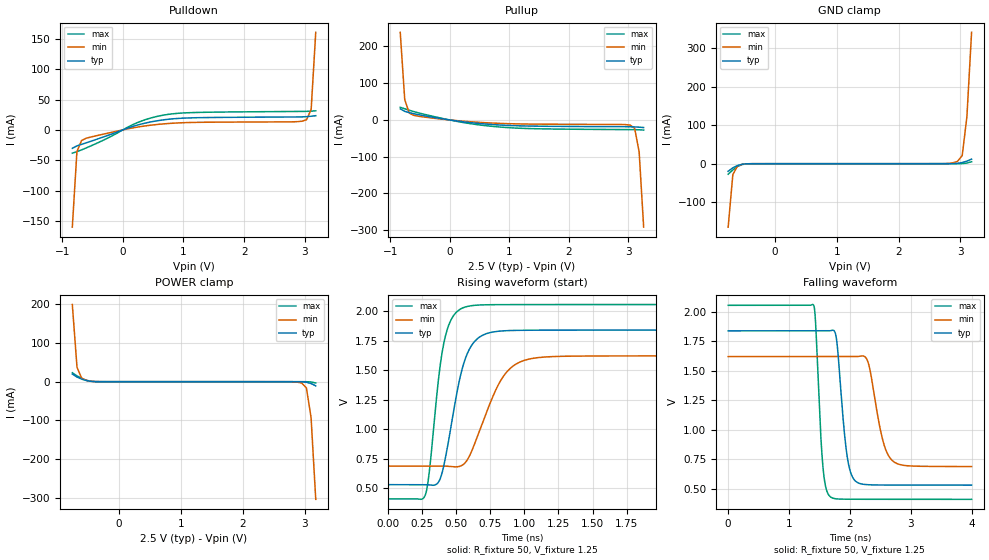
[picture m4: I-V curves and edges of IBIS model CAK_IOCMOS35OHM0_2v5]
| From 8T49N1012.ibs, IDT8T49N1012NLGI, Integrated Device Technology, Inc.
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| 3.25758e+00   -1.33581e-02   -4.69445e-01   -6.92786e-03
| 3.33333e+00   -3.05431e-02   -6.81022e-01   -1.35814e-02
| 3.40909e+00   -1.97473e-01   -8.92821e-01   -2.11713e-02
| 3.48485e+00   -4.80532e-01   -1.10478e+00   -2.82326e-02
| 3.56061e+00   -7.63803e-01   -1.31687e+00   -5.48408e-02
| 3.63636e+00   -1.04727e+00   -1.52909e+00   -3.40378e-01
| 3.71212e+00   -1.33091e+00   -1.74141e+00   -7.03030e-01
| 3.78788e+00   -1.61471e+00   -1.95383e+00   -1.06588e+00
| 3.86364e+00   -1.89867e+00   -2.16636e+00   -1.42892e+00
| 3.93939e+00   -2.18277e+00   -2.37898e+00   -1.79210e+00
| 4.01515e+00   -2.46699e+00   -2.59169e+00   -2.15542e+00
| 4.09091e+00   -2.75133e+00   -2.80449e+00   -2.51885e+00
| 4.16667e+00   -3.03577e+00   -3.01738e+00   -2.88238e+00
| 4.24242e+00   -3.32030e+00   -3.23034e+00   -3.24599e+00
| 4.31818e+00   -3.60492e+00   -3.44338e+00   -3.60966e+00
| 4.39394e+00   -3.88961e+00   -3.65649e+00   -3.97340e+00
| 4.46970e+00   -4.17436e+00   -3.86967e+00   -4.33720e+00
| 4.54545e+00   -4.45918e+00   -4.08291e+00   -4.70105e+00
| 4.62121e+00   -4.74404e+00   -4.29621e+00   -5.06495e+00
| 4.69697e+00   -5.02895e+00   -4.50957e+00   -5.42889e+00
| 4.77273e+00   -5.31390e+00   -4.72298e+00   -5.79286e+00
| 4.84848e+00   -5.59889e+00   -4.93644e+00   -6.15686e+00
| 4.92424e+00   -5.88390e+00   -5.14994e+00   -6.52088e+00
| 5.00000e+00   -6.16895e+00   -5.36349e+00   -6.88491e+00
[Model] CAK_IOCMOS35OHM0_2v5
Model_type   I/O
Polarity   Non-Inverting
|   typ   min   max
C_comp   2pF   1.5pF   2.5pF
|Input
Vinl = 0.7V
Vinh = 1.7V
|Output
Vmeas = 1.25V
Rref = 50
Cref = 0
Vref = 1.25V
|   typ   min   max
[Voltage range]   2.5V   2.375V   2.625V
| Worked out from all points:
|   slope of the pulldown table from 0 to 0.375 V, typ, clamps not added: 33.2 ohm
|   slope of the pullup table from 0 to 0.375 V, typ, clamps not added: 48.8 ohm
|   GND clamp passes 1 mA (typ) near -0.50 V on its own axis
|   POWER clamp passes 1 mA (typ) near -0.46 V on its own axis
|   rising waveform, R_fixture 50, V_fixture 1.25: 20-80 % time 134ps typ, 204ps min, 96.8ps max; typ from 0.531 V to 1.84 V
|   falling waveform, R_fixture 50, V_fixture 1.25: 20-80 % time 134ps typ, 204ps min, 95ps max; typ from 1.84 V to 0.531 V
[GND_clamp]
|Voltage   I (typ)   I (min)   I (max)
|Note, modeling breaks down at 250mA and above.  This is well beyond the functional   |
|operating range of the device.  Should this scenario occur, catastrophic failure and   |
|possible damage to the device and/or board is of higher concern than the I-V curve   |
|behavior.  The IBIS checker will flag currents in excess of 10A with warnings.  Lines   |
|with currents in excess of 0.35 A have been commented out.  The points still remain|
|available to the user if the user desires to use them.   |
|-2.42424e+00   -5.99088e+00   -4.88415e+00   -7.24880e+00
|-2.34848e+00   -5.70272e+00   -4.66840e+00   -6.88094e+00
|-2.27273e+00   -5.41462e+00   -4.45272e+00   -6.51310e+00
|-2.19697e+00   -5.12656e+00   -4.23712e+00   -6.14529e+00
|-2.12121e+00   -4.83856e+00   -4.02161e+00   -5.77750e+00
|-2.04545e+00   -4.55064e+00   -3.80620e+00   -5.40975e+00
|-1.96970e+00   -4.26278e+00   -3.59088e+00   -5.04205e+00
|-1.89394e+00   -3.97502e+00   -3.37567e+00   -4.67441e+00
|-1.81818e+00   -3.68735e+00   -3.16057e+00   -4.30683e+00
|-1.74242e+00   -3.39979e+00   -2.94558e+00   -3.93934e+00
|-1.66667e+00   -3.11235e+00   -2.73072e+00   -3.57193e+00
|-1.59091e+00   -2.82505e+00   -2.51599e+00   -3.20462e+00
|-1.51515e+00   -2.53790e+00   -2.30139e+00   -2.83743e+00
|-1.43939e+00   -2.25092e+00   -2.08694e+00   -2.47036e+00
|-1.36364e+00   -1.96413e+00   -1.87263e+00   -2.10344e+00
|-1.28788e+00   -1.67754e+00   -1.65847e+00   -1.73670e+00
|-1.21212e+00   -1.39118e+00   -1.44447e+00   -1.37017e+00
|-1.13636e+00   -1.10506e+00   -1.23064e+00   -1.00389e+00
|-1.06061e+00   -8.19198e-01   -1.01701e+00   -6.37879e-01
|-9.84848e-01   -5.33627e-01   -8.03591e-01   -2.72184e-01
|-9.09091e-01   -2.48371e-01   -5.90465e-01   -5.58283e-02
|-8.33333e-01   -4.53732e-02   -3.77762e-01   -3.79192e-02
-757.6mV  -19.7mA    -165.1mA   -27.4mA
-681.8mV  -10.83mA   -28.37mA   -16.29mA
-606.1mV  -4.786mA   -6.047mA   -7.399mA
-530.3mV  -1.407mA   -1.506mA   -2.105mA
-378.8mV  -80.75uA   -97.08uA   -91.06uA
2.727V    4.903uA    107uA      2.354uA
2.879V    114.3uA    2.196mA    6.393uA
2.955V    801.8uA    6.121mA    22.36uA
3.03V     2.877mA    21.15mA    238.2uA
3.106V    6.558mA    121.9mA    1.646mA
3.182V    11.89mA    341.6mA    5.038mA
| 3.25758e+00   1.96472e-02   5.60110e-01   1.04123e-02
| 3.33333e+00   4.87507e-02   7.78570e-01   1.76749e-02
| 3.40909e+00   2.77107e-01   9.97201e-01   2.56783e-02
| 3.48485e+00   5.68788e-01   1.21604e+00   3.28468e-02
| 3.56061e+00   8.60732e-01   1.43508e+00   7.83400e-02
| 3.63636e+00   1.15296e+00   1.65434e+00   4.20975e-01
| 3.71212e+00   1.44548e+00   1.87382e+00   7.94432e-01
| 3.78788e+00   1.73828e+00   2.09351e+00   1.16825e+00
| 3.86364e+00   2.03137e+00   2.31341e+00   1.54243e+00
| 3.93939e+00   2.32473e+00   2.53352e+00   1.91695e+00
| 4.01515e+00   2.61836e+00   2.75385e+00   2.29181e+00
| 4.09091e+00   2.91225e+00   2.97438e+00   2.66701e+00
| 4.16667e+00   3.20641e+00   3.19513e+00   3.04252e+00
| 4.24242e+00   3.50082e+00   3.41608e+00   3.41834e+00
| 4.31818e+00   3.79548e+00   3.63725e+00   3.79446e+00
| 4.39394e+00   4.09039e+00   3.85863e+00   4.17087e+00
| 4.46970e+00   4.38554e+00   4.08023e+00   4.54756e+00
| 4.54545e+00   4.68094e+00   4.30204e+00   4.92452e+00
| 4.62121e+00   4.97658e+00   4.52407e+00   5.30175e+00
| 4.69697e+00   5.27245e+00   4.74633e+00   5.67924e+00
| 4.77273e+00   5.56857e+00   4.96881e+00   6.05699e+00
| 4.84848e+00   5.86492e+00   5.19152e+00   6.43499e+00
| 4.92424e+00   6.16151e+00   5.41446e+00   6.81323e+00
| 5.00000e+00   6.45834e+00   5.63765e+00   7.19172e+00
[Power_clamp]
|Voltage   I (typ)   I (min)   I (max)
|Note, modeling breaks down at 250mA and above.  This is well beyond the functional   |
|operating range of the device.  Should this scenario occur, catastrophic failure and   |
|possible damage to the device and/or board is of higher concern than the I-V curve   |
|behavior.  The IBIS checker will flag currents in excess of 10A with warnings.  Lines   |
|with currents in excess of 0.35 A have been commented out.  The points still remain|
|available to the user if the user desires to use them.   |
|-2.42424e+00   6.16151e+00   5.04673e+00   7.43787e+00
|-2.34848e+00   5.86492e+00   4.82417e+00   7.05922e+00
|-2.27273e+00   5.56857e+00   4.60184e+00   6.68082e+00
|-2.19697e+00   5.27245e+00   4.37973e+00   6.30266e+00
|-2.12121e+00   4.97658e+00   4.15784e+00   5.92475e+00
|-2.04545e+00   4.68094e+00   3.93617e+00   5.54709e+00
|-1.96970e+00   4.38554e+00   3.71471e+00   5.16969e+00
|-1.89394e+00   4.09039e+00   3.49347e+00   4.79255e+00
|-1.81818e+00   3.79548e+00   3.27244e+00   4.41568e+00
|-1.74242e+00   3.50082e+00   3.05162e+00   4.03909e+00
|-1.66667e+00   3.20641e+00   2.83101e+00   3.66278e+00
|-1.59091e+00   2.91225e+00   2.61061e+00   3.28677e+00
|-1.51515e+00   2.61836e+00   2.39042e+00   2.91105e+00
|-1.43939e+00   2.32473e+00   2.17045e+00   2.53565e+00
|-1.36364e+00   2.03137e+00   1.95069e+00   2.16057e+00
|-1.28788e+00   1.73828e+00   1.73114e+00   1.78583e+00
|-1.21212e+00   1.44548e+00   1.51180e+00   1.41142e+00
|-1.13636e+00   1.15296e+00   1.29268e+00   1.03737e+00
|-1.06061e+00   8.60732e-01   1.07377e+00   6.63681e-01
|-9.84848e-01   5.68788e-01   8.55069e-01   2.90350e-01
|-9.09091e-01   2.77107e-01   6.36557e-01   4.68087e-02
|-8.33333e-01   4.87507e-02   4.18123e-01   3.00765e-02
-757.6mV  19.65mA    199mA      23mA
-681.8mV  11.89mA    37.01mA    14.94mA
-606.1mV  6.558mA    8.981mA    8.308mA
-530.3mV  2.877mA    3.169mA    3.622mA
-303mV    14.46uA    30.61uA    12.18uA
2.727V    -54.42uA   -72.56uA   -62.76uA
2.879V    -80.75uA   -908.8uA   -66.34uA
2.955V    -281.2uA   -3.717mA   -70.88uA
3.03V     -1.407mA   -15.93mA   -127.8uA
3.106V    -4.786mA   -92.25mA   -684.1uA
3.182V    -10.83mA   -303.4mA   -3.499mA
| 3.25758e+00   -1.96989e-02   -5.15962e-01   -1.01554e-02
| 3.33333e+00   -4.53732e-02   -7.28958e-01   -2.00234e-02
| 3.40909e+00   -2.48371e-01   -9.42283e-01   -3.12866e-02
| 3.48485e+00   -5.33627e-01   -1.15585e+00   -4.17513e-02
| 3.56061e+00   -8.19198e-01   -1.36961e+00   -8.15325e-02
| 3.63636e+00   -1.10506e+00   -1.58355e+00   -4.00139e-01
| 3.71212e+00   -1.39118e+00   -1.79765e+00   -7.65947e-01
| 3.78788e+00   -1.67754e+00   -2.01191e+00   -1.13206e+00
| 3.86364e+00   -1.96413e+00   -2.22632e+00   -1.49843e+00
| 3.93939e+00   -2.25092e+00   -2.44086e+00   -1.86504e+00
| 4.01515e+00   -2.53790e+00   -2.65555e+00   -2.23184e+00
| 4.09091e+00   -2.82505e+00   -2.87037e+00   -2.59881e+00
| 4.16667e+00   -3.11235e+00   -3.08531e+00   -2.96593e+00
| 4.24242e+00   -3.39979e+00   -3.30037e+00   -3.33317e+00
| 4.31818e+00   -3.68735e+00   -3.51555e+00   -3.70052e+00
| 4.39394e+00   -3.97502e+00   -3.73083e+00   -4.06795e+00
| 4.46970e+00   -4.26278e+00   -3.94621e+00   -4.43548e+00
| 4.54545e+00   -4.55064e+00   -4.16168e+00   -4.80307e+00
| 4.62121e+00   -4.83856e+00   -4.37725e+00   -5.17074e+00
| 4.69697e+00   -5.12656e+00   -4.59290e+00   -5.53846e+00
| 4.77273e+00   -5.41462e+00   -4.80863e+00   -5.90622e+00
| 4.84848e+00   -5.70272e+00   -5.02443e+00   -6.27402e+00
| 4.92424e+00   -5.99088e+00   -5.24031e+00   -6.64184e+00
| 5.00000e+00   -6.27908e+00   -5.45625e+00   -7.00969e+00
[Pulldown]
|Voltage   I (typ)   I (min)   I (max)
|Note, modeling breaks down at 250mA and above.  This is well beyond the functional   |
|operating range of the device.  Should this scenario occur, catastrophic failure and   |
|possible damage to the device and/or board is of higher concern than the I-V curve   |
|behavior.  The IBIS checker will flag currents in excess of 10A with warnings.  Lines   |
|with currents in excess of 0.35 A have been commented out.  The points still remain|
|available to the user if the user desires to use them.   |
|-2.424240e+00   -5.620920e+00   -4.561270e+00   -6.831600e+00
|-2.348480e+00   -5.341380e+00   -4.351820e+00   -6.474360e+00
|-2.272730e+00   -5.061780e+00   -4.142370e+00   -6.117000e+00
|-2.196970e+00   -4.782250e+00   -3.932930e+00   -5.759610e+00
|-2.121210e+00   -4.502700e+00   -3.723470e+00   -5.402300e+00
|-2.045450e+00   -4.223130e+00   -3.514010e+00   -5.044950e+00
|-1.969700e+00   -3.943570e+00   -3.304540e+00   -4.687600e+00
|-1.893940e+00   -3.663980e+00   -3.095070e+00   -4.330220e+00
|-1.818180e+00   -3.384390e+00   -2.885580e+00   -3.972840e+00
|-1.742420e+00   -3.104780e+00   -2.676080e+00   -3.615430e+00
|-1.666670e+00   -2.825150e+00   -2.466570e+00   -3.258010e+00
|-1.590910e+00   -2.545490e+00   -2.257030e+00   -2.900560e+00
|-1.515150e+00   -2.265810e+00   -2.047480e+00   -2.543070e+00
|-1.439390e+00   -1.986090e+00   -1.837900e+00   -2.185550e+00
|-1.363640e+00   -1.706320e+00   -1.628300e+00   -1.827980e+00
|-1.287880e+00   -1.426520e+00   -1.418670e+00   -1.470360e+00
|-1.212120e+00   -1.146650e+00   -1.209020e+00   -1.112660e+00
|-1.136360e+00   -8.667200e-01   -9.993300e-01   -7.548700e-01
|-1.060610e+00   -5.867220e-01   -7.896000e-01   -3.969910e-01
|-9.848480e-01   -3.066460e-01   -5.798390e-01   -7.806800e-02
|-9.090910e-01   -6.551900e-02   -3.700490e-01   -4.152980e-02
-833.3mV  -30.4mA    -160.2mA   -38.37mA
-757.6mV  -26.34mA   -35.84mA   -35.89mA
-681.8mV  -23.84mA   -17.61mA   -32.95mA
-606.1mV  -21.34mA   -13.8mA    -29.8mA
227.3mV   7.551mA    4.361mA    11.42mA
454.5mV   12.99mA    7.63mA     19.37mA
681.8mV   16.67mA    9.951mA    24.52mA
1.212V    20.01mA    12.36mA    28.66mA
2.803V    21.22mA    13.27mA    30.3mA
3.03V     21.8mA     16.76mA    30.5mA
3.106V    22.45mA    33.64mA    30.79mA
3.182V    23.38mA    160.7mA    31.41mA
|3.257580e+00   2.470960e-02   3.762400e-01   3.236290e-02
|3.333330e+00   2.959920e-02   5.918100e-01   3.363400e-02
|3.409090e+00   1.001510e-01   8.074090e-01   3.503170e-02
|3.484850e+00   3.838970e-01   1.023030e+00   3.629400e-02
|3.560610e+00   6.718180e-01   1.238710e+00   4.394800e-02
|3.636360e+00   9.597900e-01   1.454410e+00   2.364620e-01
|3.712120e+00   1.247810e+00   1.670150e+00   6.046980e-01
|3.787880e+00   1.535890e+00   1.885920e+00   9.730100e-01
|3.863640e+00   1.824010e+00   2.101740e+00   1.341380e+00
|3.939390e+00   2.112190e+00   2.317600e+00   1.709840e+00
|4.015150e+00   2.400420e+00   2.533480e+00   2.078370e+00
|4.090910e+00   2.688710e+00   2.749420e+00   2.446960e+00
|4.166670e+00   2.977050e+00   2.965390e+00   2.815630e+00
|4.242420e+00   3.265440e+00   3.181400e+00   3.184380e+00
|4.318180e+00   3.553900e+00   3.397450e+00   3.553210e+00
|4.393940e+00   3.842420e+00   3.613550e+00   3.922130e+00
|4.469700e+00   4.131000e+00   3.829690e+00   4.291130e+00
|4.545450e+00   4.419630e+00   4.045870e+00   4.660220e+00
|4.621210e+00   4.708340e+00   4.262110e+00   5.029450e+00
|4.696970e+00   4.997150e+00   4.478390e+00   5.398660e+00
|4.772730e+00   5.285930e+00   4.694720e+00   5.768110e+00
|4.848480e+00   5.574880e+00   4.911080e+00   6.137610e+00
|4.924240e+00   5.863890e+00   5.127540e+00   6.507170e+00
|5.000000e+00   6.153060e+00   5.344050e+00   6.876880e+00
[Pullup]
|Voltage   I (typ)   I (min)   I (max)
|Note, modeling breaks down at 250mA and above.  This is well beyond the functional   |
|operating range of the device.  Should this scenario occur, catastrophic failure and   |
|possible damage to the device and/or board is of higher concern than the I-V curve   |
|behavior.  The IBIS checker will flag currents in excess of 10A with warnings.  Lines   |
|with currents in excess of 0.35 A have been commented out.  The points still remain|
|available to the user if the user desires to use them.   |
|-2.424240e+00   5.884990e+00   4.790360e+00   7.136830e+00
|-2.348480e+00   5.595580e+00   4.573450e+00   6.766980e+00
|-2.272730e+00   5.306130e+00   4.356560e+00   6.397080e+00
|-2.196970e+00   5.016750e+00   4.139690e+00   6.027240e+00
|-2.121210e+00   4.727390e+00   3.922850e+00   5.657350e+00
|-2.045450e+00   4.438030e+00   3.706020e+00   5.287510e+00
|-1.969700e+00   4.148680e+00   3.489220e+00   4.917710e+00
|-1.893940e+00   3.859340e+00   3.272430e+00   4.547940e+00
|-1.818180e+00   3.570020e+00   3.055660e+00   4.178140e+00
|-1.742420e+00   3.280710e+00   2.838900e+00   3.808350e+00
|-1.666670e+00   2.991410e+00   2.622170e+00   3.438570e+00
|-1.590910e+00   2.702130e+00   2.405450e+00   3.068780e+00
|-1.515150e+00   2.412850e+00   2.188750e+00   2.699010e+00
|-1.439390e+00   2.123580e+00   1.972050e+00   2.329220e+00
|-1.363640e+00   1.834310e+00   1.755360e+00   1.959430e+00
|-1.287880e+00   1.545050e+00   1.538690e+00   1.589620e+00
|-1.212120e+00   1.255770e+00   1.322030e+00   1.219810e+00
|-1.136360e+00   9.665000e-01   1.105370e+00   8.499700e-01
|-1.060610e+00   6.772080e-01   8.887100e-01   4.801090e-01
|-9.848480e-01   3.878980e-01   6.720410e-01   1.143440e-01
|-9.090910e-01   1.026590e-01   4.553330e-01   3.942970e-02
-833.3mV  30.43mA    238.5mA    34.47mA
-757.6mV  23.4mA     55.15mA    30.53mA
-681.8mV  19.94mA    18.68mA    26.41mA
-606.1mV  17.11mA    12.63mA    22.8mA
151.5mV   -3.441mA   -2.312mA   -4.819mA
833.3mV   -13.62mA   -9.198mA   -19.09mA
1.439V    -16.78mA   -11.29mA   -23.78mA
2.955V    -18.33mA   -12.6mA    -26.15mA
3.03V     -18.49mA   -13.96mA   -26.22mA
3.106V    -18.9mA    -22.45mA   -26.34mA
3.182V    -19.59mA   -87.06mA   -26.7mA
3.258V    -20.6mA    -291.6mA   -27.48mA
|3.333330e+00   -2.346490e-02   -5.006320e-01   -2.861170e-02
|3.409090e+00   -5.753200e-02   -7.096670e-01   -2.989430e-02
|3.484850e+00   -2.977200e-01   -9.187300e-01   -3.108580e-02
|3.560610e+00   -5.769620e-01   -1.127830e+00   -3.553250e-02
|3.636360e+00   -8.562400e-01   -1.336930e+00   -1.541430e-01
|3.712120e+00   -1.135550e+00   -1.546060e+00   -5.113230e-01
|3.787880e+00   -1.414880e+00   -1.755200e+00   -8.685300e-01
|3.863640e+00   -1.694240e+00   -1.964350e+00   -1.225770e+00
|3.939390e+00   -1.973620e+00   -2.173530e+00   -1.583030e+00
|4.015150e+00   -2.253020e+00   -2.382720e+00   -1.940320e+00
|4.090910e+00   -2.532440e+00   -2.591920e+00   -2.297640e+00
|4.166670e+00   -2.811880e+00   -2.801140e+00   -2.654970e+00
|4.242420e+00   -3.091330e+00   -3.010380e+00   -3.012320e+00
|4.318180e+00   -3.370810e+00   -3.219620e+00   -3.369680e+00
|4.393940e+00   -3.650300e+00   -3.428890e+00   -3.727080e+00
|4.469700e+00   -3.929810e+00   -3.638170e+00   -4.084480e+00
|4.545450e+00   -4.209330e+00   -3.847470e+00   -4.441910e+00
|4.621210e+00   -4.488880e+00   -4.056780e+00   -4.799350e+00
|4.696970e+00   -4.768440e+00   -4.266100e+00   -5.156840e+00
|4.772730e+00   -5.047980e+00   -4.475440e+00   -5.514280e+00
|4.848480e+00   -5.327580e+00   -4.684810e+00   -5.871780e+00
|4.924240e+00   -5.607220e+00   -4.894190e+00   -6.229360e+00
|5.000000e+00   -5.886920e+00   -5.103550e+00   -6.586910e+00
[Ramp]
|   typ   min   max
dV/dt_r   0.788/0.134n   0.563/0.205n   0.989/0.096n
dV/dt_f   0.788/0.134n   0.562/0.204n   0.991/0.095n
R_load =   50
[Rising Waveform]
R_fixture = 50
V_fixture = 1.25   |Vcc_typ
V_fixture_min = 1.1875 |Vcc_min
V_fixture_max = 1.3125 |Vcc_max
C_fixture = 0.0p
| Time   typ   min   max
0s        531.3mV    688.6mV    411mV
271.1ps   531.5mV    688.6mV    438.6mV
302.2ps   529.7mV    688.7mV    637.4mV
360ps     539.7mV    689mV      1.318V
408.9ps   692.4mV    688.6mV    1.728V
560ps     1.575V     710.4mV    2.033V
657.8ps   1.769V     946.1mV    2.051V
831.1ps   1.832V     1.422V     2.055V
1.031ns   1.838V     1.593V     2.056V
4ns       1.84V      1.621V     2.056V
[Falling Waveform]
R_fixture = 50
V_fixture = 1.25   |Vcc_typ
V_fixture_min = 1.1875 |Vcc_min
V_fixture_max = 1.3125 |Vcc_max
C_fixture = 0.0p
| Time   typ   min   max
0s        1.84V      1.621V     2.056V
1.404ns   1.84V      1.621V     2.057V
1.556ns   1.84V      1.621V     697.3mV
1.68ns    1.841V     1.621V     432mV
1.778ns   1.778V     1.621V     415.1mV
1.942ns   824.5mV    1.621V     412mV
2.08ns    572.1mV    1.621V     411.6mV
2.293ns   535mV      1.581V     411.3mV
2.698ns   531.9mV    739.8mV    411.1mV
4ns       531.4mV    688.9mV    411mV
